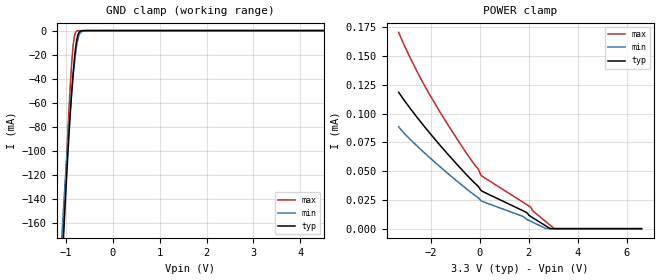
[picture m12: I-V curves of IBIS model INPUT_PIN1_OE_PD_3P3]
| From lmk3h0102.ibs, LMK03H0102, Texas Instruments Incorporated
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[Model]   INPUT_PIN1_OE_PD_3P3
Model_type   Input
Vinl = 0.65
Vinh = 1.15
|   typ   min   max
C_comp   0.7pF   0.5pF   0.9pF
[Voltage Range]   3.3   3.135   3.465
[Temperature Range]   45   125   -40
[Power Clamp Reference]   3.3   3.135   3.465
[GND Clamp Reference]   0   0   0
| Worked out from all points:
|   GND clamp passes 1 mA (typ) near -0.71 V on its own axis
[GND Clamp]
|   Voltage   I(typ)   I(min)   I(max)
-3.3V     -2.163A    -1.946A    -2.393A
-1.142V   -244.3mA   -209.2mA   -247.1mA
-1.073V   -188.3mA   -161.6mA   -183.1mA
-1.043V   -165mA     -142.2mA   -156.3mA
-943.8mV  -92.69mA   -84.35mA   -72.63mA
-874.5mV  -50.33mA   -50.21mA   -25.69mA
-844.8mV  -35.17mA   -37.37mA   -12.01mA
-815.1mV  -22.23mA   -25.95mA   -4.039mA
-765.6mV  -7.235mA   -11.31mA   -401.3uA
-696.3mV  -683.6uA   -2.04mA    -32.8uA
-577.5mV  -20.36uA   -85.13uA   -17.77uA
6.6V      0A         0A         0A
[POWER Clamp]
|   Voltage   I(typ)   I(min)   I(max)
-3.3V     118.6uA    88.59uA    170.7uA
-2.805V   103.9uA    77.12uA    147.5uA
-1.954V   81.1uA     60.24uA    113.5uA
-1.231V   63.2uA     46.83uA    88.29uA
-62.7mV   36.89uA    26.95uA    51.9uA
85.8mV    32.82uA    23.98uA    45.9uA
1.888V    14.29uA    8.546uA    21.37uA
2.046V    11.07uA    6.787uA    19.18uA
2.175V    9.322uA    5.468uA    15.42uA
2.709V    2.209uA    5.923nA    5.897uA
3.036V    0A         0A         112.6nA
6.6V      0A         0A         0A
